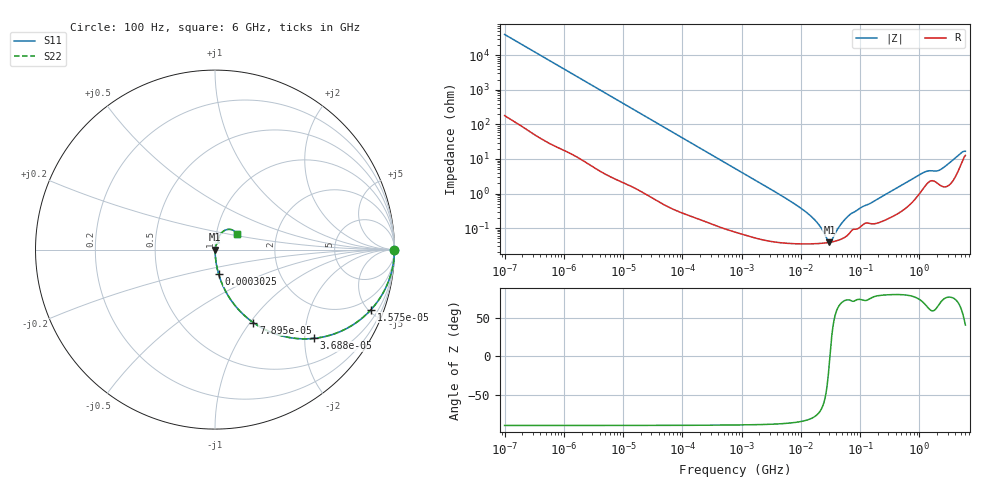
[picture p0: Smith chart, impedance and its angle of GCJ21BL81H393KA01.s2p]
!Murata Part Number: GCJ21BL81H393KA01
!These Parameters are Measured in Series Mode Connection
!Data Generated on Mar 13, 2026
!  o--ll--o
!Port1  Port2
!  o------o
!Operation Temp=25[degC], DC Bias Voltage=0[V]
!Freq. Start=100[Hz] Stop=6[GHz] 401[Steps]
# Hz S RI R 50
!Freq.(Hz) S11(Real) S11(Imag) S21(Real) S21(Imag) S12(Real) S12(Imag) S22(Real) S22(Imag)
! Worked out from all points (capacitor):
!   401 points, 100 Hz to 6 GHz, reference 50 ohm
!   read as one part in series: C = 39.5 nF near 109 Hz
!   lowest |Z| = 38.9 mohm at 30.45 MHz (marker M1)
!   series resonance near 31.01 MHz, so ESL is about 670 pH
!   S11 on the Smith chart (normalised r, x): 100 Hz: open; 15.75 kHz: 1.03, -5.18; 36.88 kHz: 1.01, -2.22; 78.95 kHz: 1.01, -1.04; 302.5 kHz: 1.00, -0.27; 6 GHz: 1.25, +0.22
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100  1 -0.00249  1.73e-05 0.00249  1.73e-05 0.00249  1 -0.00249
2008  0.9973 -0.0494  0.00267 0.0494  0.00267 0.0494  0.9973 -0.0494
6151  0.977 -0.1476  0.023 0.1476  0.023 0.1476  0.977 -0.1476
15752  0.8689 -0.3347  0.1311 0.3347  0.1311 0.3347  0.8689 -0.3347
36880  0.5517 -0.4945  0.4483 0.4945  0.4483 0.4945  0.5517 -0.4945
40335  0.5075 -0.4971  0.4925 0.4971  0.4925 0.4971  0.5075 -0.4971
78952  0.214 -0.4071  0.786 0.4071  0.786 0.4071  0.214 -0.4071
141303  0.0797 -0.2671  0.9203 0.2671  0.9203 0.2671  0.0797 -0.2671
302498  0.0195 -0.1335  0.9805 0.1335  0.9805 0.1335  0.0195 -0.1335
774597  0.00361 -0.0533  0.9964 0.0533  0.9964 0.0533  0.00361 -0.0533
6644369  0.000394 -0.00601  0.9996 0.00601  0.9996 0.00601  0.000394 -0.00601
1.555665e7  0.000354 -0.00202  0.9996 0.00202  0.9996 0.00202  0.000354 -0.00202
2.035112e7  0.000359 -0.00117  0.9996 0.00117  0.9996 0.00117  0.000359 -0.00117
3.045065e7  0.000386 -4.87e-05  0.9996 4.87e-05  0.9996 4.87e-05  0.000386 -4.87e-05
3.330331e7  0.000397 0.000194  0.9996 -0.000194  0.9996 -0.000194  0.000397 0.000194
4.983056e7  0.000492 0.00135  0.9995 -0.00135  0.9995 -0.00135  0.000492 0.00135
6.817316e7  0.000756 0.00238  0.9992 -0.00238  0.9992 -0.00238  0.000756 0.00238
3.124326e8  0.00205 0.0106  0.998 -0.0106  0.998 -0.0106  0.00205 0.0106
1.197065e9  0.016 0.0371  0.984 -0.0371  0.984 -0.0371  0.016 0.0371
2.240541e9  0.0191 0.0437  0.9809 -0.0437  0.9809 -0.0437  0.0191 0.0437
4.796499e9  0.0663 0.1116  0.9337 -0.1116  0.9337 -0.1116  0.0663 0.1116
6e9  0.1209 0.0845  0.8791 -0.0845  0.8791 -0.0845  0.1209 0.0845
